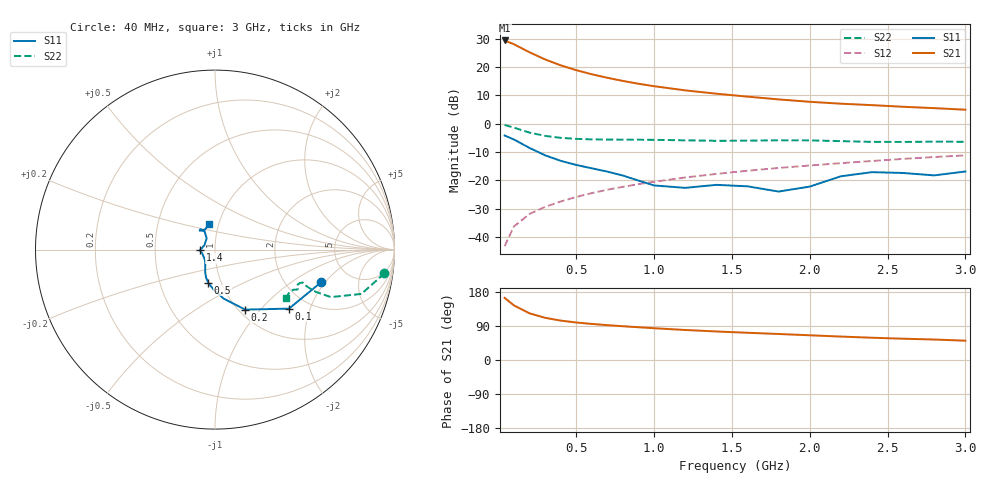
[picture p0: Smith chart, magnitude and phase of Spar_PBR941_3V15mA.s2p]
! Filename:  PBR941F.S2P  Version:  3.0
! NXP part #:  PBR941  Date: July 1998
! Bias condition:  Vce=3V, Ic=15mA
#  MHz  S  MA  R 50
! Freq  S11  S21  S12  S22
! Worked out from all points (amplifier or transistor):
!   21 points, 40 MHz to 3 GHz, reference 50 ohm
!   highest |S21| = 29.3 dB at 40 MHz (marker M1)
!   |S21| within 3 dB of that: start of sweep to 158.7 MHz
!   unconditionally stable (mu >= 1): 804.3 MHz to 2.264 GHz
!   at 300 MHz: K = 0.81, MSG = 26.0 dB, |S12| = -29.3 dB
!   at 1 GHz: K = 1.02, MAG = 16.0 dB, |S12| = -20.4 dB
!   at 3 GHz: K = 0.98, MSG = 8.1 dB, |S12| = -11.2 dB
!   S11 on the Smith chart (normalised r, x): 40 MHz: 3.11, -1.82; 100 MHz: 1.59, -1.45; 200 MHz: 1.07, -0.83; 500 MHz: 0.87, -0.33; 1.4 GHz: 0.85, -0.01; 3 GHz: 0.90, +0.26
40  0.6198 -16.9  29.3 163.9  0.006961 80.7  0.9531 -8.0
100  0.5275 -38.6  25.12 144.0  0.0155 75.1  0.8523 -16.8
200  0.3743 -63.3  18.13 123.1  0.02573 71.2  0.6975 -22.3
300  0.2777 -79.9  13.58 111.4  0.03429 72.3  0.6103 -22.8
400  0.2221 -92.2  10.68 104.0  0.04258 73.7  0.5645 -22.1
500  0.1878 -101.6  8.782 98.9  0.0512 75.5  0.541 -21.6
600  0.1639 -107.6  7.437 95.2  0.05986 76.1  0.5296 -21.1
700  0.1432 -112.1  6.441 92.0  0.06876 77.3  0.5252 -20.9
800  0.1221 -116.8  5.671 89.1  0.07717 77.6  0.5239 -20.7
900  0.09965 -122.8  5.061 86.4  0.08615 78.3  0.5227 -20.6
1000  0.08179 -133.2  4.583 83.9  0.09496 78.2  0.52 -20.7
1200  0.07409 -163.2  3.868 79.2  0.1129 78.3  0.5097 -21.4
1400  0.08376 -177.4  3.381 75.3  0.1304 77.9  0.5002 -22.9
1600  0.0789 178.3  3 71.9  0.1484 77.9  0.5024 -24.4
1800  0.0638 157.9  2.681 68.6  0.1662 77.6  0.5106 -25.4
2000  0.07807 126.3  2.434 65.2  0.1837 76.8  0.5088 -26.0
2200  0.1187 119.7  2.252 61.8  0.202 75.9  0.4934 -26.9
2400  0.1401 125.4  2.125 58.8  0.2205 75.2  0.4788 -29.1
2600  0.1356 129.0  1.988 56.2  0.2402 74.8  0.4774 -31.9
2800  0.1229 119.5  1.881 54.0  0.2593 74.1  0.4836 -33.8
3000  0.1439 103.0  1.766 51.0  0.2766 72.9  0.4801 -34.4
